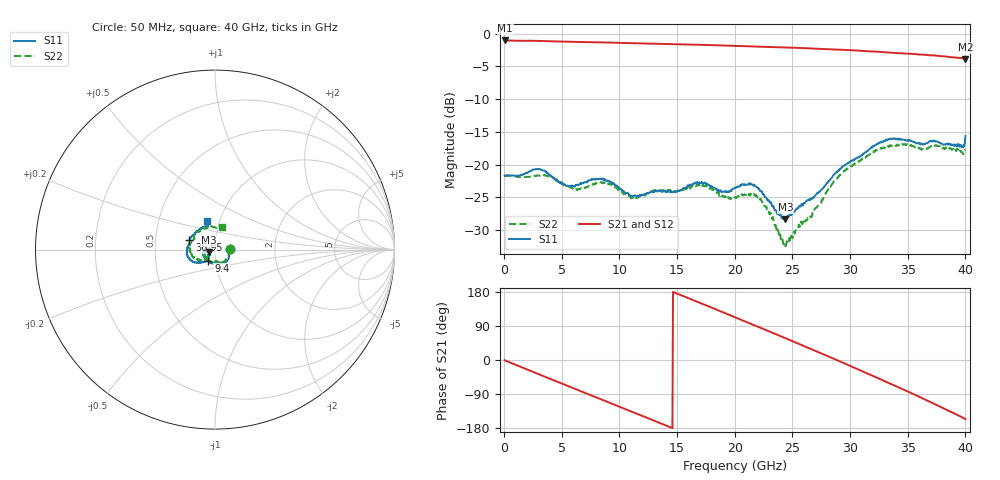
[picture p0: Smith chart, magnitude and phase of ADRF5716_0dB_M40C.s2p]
! Device: ADRF5716
! Description: 30GHz 2-Bit Digital Attenuator
! Frequency: 100 MHz – 30 GHz
! Ports:
! ATTIN  = Port 1
! ATTOUT = Port 2
! State: 0 dB Attenuation selected
! Supply Voltage:
! VDD  =  +3.30 Volts
! VSS  =  -3.30 Volts
! Control Voltages:
! D5 = 0V, D6 = 0V
! Temperature = -40 C
! Data: Data was collected using a calibrated network analyzer.
!  The reference plane is the package pins of ADRF5716 switch.
! Note: Analog Devices supplies this data as a sample of measured data for this product.
!  Your particular data for this product may vary.
!  Analog Devices reserves the right to change this data at anytime
# HZ S DB R 50
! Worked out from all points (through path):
!   800 points, 50 MHz to 40 GHz, reference 50 ohm
!   highest |S21| = -1.05 dB at 100 MHz (marker M1); lowest = -3.9 dB at 40 GHz (marker M2)
!   group delay of S21, straight-line fit = 35.4 ps
!   lowest |S11| = -28.4 dB at 24.4 GHz (marker M3), VSWR 1.08, Z = 46.6 - j1.47 ohm
!   |S11| at or under -10 dB: start of sweep to end of sweep
!   |S22| runs from -32.5 to -16.9 dB; largest |S21 - S12| = 0
!   S11 on the Smith chart (normalised r, x): 50 MHz: 1.18, +0.00; 9.4 GHz: 0.92, -0.12; 36.95 GHz: 0.75, +0.08; 40 GHz: 0.87, +0.29
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5e7  -21.68 1.2  -1.05 -0.6  -1.05 -0.6  -21.74 2.2
1e8  -21.64 -1.3  -1.05 -1.4  -1.05 -1.4  -21.71 -1.3
3e9  -20.71 -46.0  -1.12 -37.3  -1.12 -37.3  -21.66 -43.9
4.85e9  -22.72 -75.1  -1.22 -60.2  -1.22 -60.2  -22.59 -74.1
6.75e9  -22.89 -85.5  -1.30 -83.4  -1.30 -83.4  -23.68 -86.6
9.4e9  -22.74 -119.9  -1.38 -115.9  -1.38 -115.9  -23.16 -118.1
1.115e10  -24.80 -126.1  -1.47 -137.3  -1.47 -137.3  -25.09 -125.9
1.34e10  -24.01 -132.0  -1.56 -164.9  -1.56 -164.9  -23.83 -134.7
1.495e10  -24.10 -135.9  -1.62 175.9  -1.62 175.9  -24.18 -142.6
1.655e10  -22.83 -142.9  -1.70 156.3  -1.70 156.3  -23.24 -151.1
1.84e10  -23.65 -155.9  -1.79 133.2  -1.79 133.2  -24.10 -168.3
2.005e10  -23.48 -153.3  -1.87 112.4  -1.87 112.4  -24.98 -167.0
2.205e10  -23.74 -170.7  -1.99 87.4  -1.99 87.4  -24.96 177.7
2.44e10  -28.36 -155.6  -2.12 57.5  -2.12 57.5  -32.47 -167.2
2.67e10  -25.26 -134.3  -2.29 27.8  -2.29 27.8  -27.83 -129.8
2.835e10  -22.17 -128.3  -2.41 6.5  -2.41 6.5  -23.25 -128.5
2.99e10  -19.70 -136.6  -2.52 -14.1  -2.52 -14.1  -20.44 -141.0
3.335e10  -16.09 -164.9  -2.89 -60.4  -2.89 -60.4  -17.32 -174.4
3.52e10  -16.29 173.4  -3.08 -85.6  -3.08 -85.6  -17.11 162.9
3.695e10  -16.38 160.2  -3.31 -110.7  -3.31 -110.7  -17.26 148.7
3.965e10  -17.38 111.4  -3.71 -150.1  -3.71 -150.1  -17.99 92.6
4e10  -15.62 105.0  -3.90 -155.9  -3.90 -155.9  -17.70 72.3
